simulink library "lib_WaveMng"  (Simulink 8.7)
settings: Solver=ode45  StartTime=0.0  StopTime=10.0  RelTol=1e-3
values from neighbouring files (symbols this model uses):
  Tstep = 0.0005    [TestOrthOscObjO_init.m]    (also in TestWaveMng_init.m = 5e-05)
undefined symbols (not defined in the file or in its folder): avgSteps, incrAvgSteps, P_WaveData_FB, P_WaveMng_FB, P_WaveMngIx_FB, stepA_WaveMngIx_FB, stepSimulink_AvgWave_FB, stepSimulink_WaveData_FB, stepSimulink_WaveMng_FB, u1, u2, void, work1, y1
libraries: lib_WaveMng x22, Lib_FunctionBlocks x6, lib_Conv x2

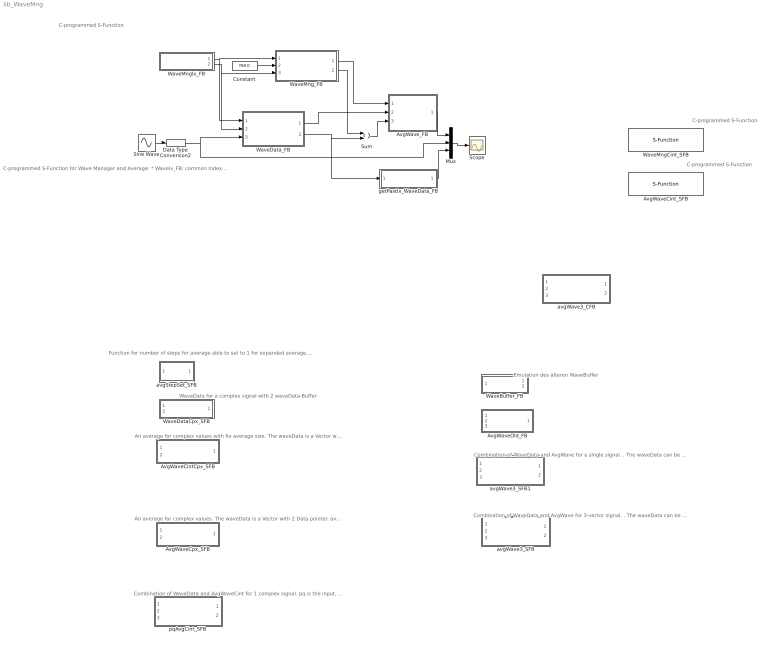
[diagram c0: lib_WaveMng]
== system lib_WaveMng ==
  note: Emulation des älteren WaveBuffer
  note: WaveData for a complex signal with 2 waveData-Buffer
  note: Function for number of steps for average able to set to 1 for expanded average. Parameter avgSteps
  note: C-programmed S-Function
  note: Combination of WaveData and AvgWaveCint for 1 complex signal. pq is the input, avg is the output. The waveData can be used for other accesses. It is a vector o2 2 pointer.
  note: An average for complex values. The waveData is a Vector with 2 Data pointer. avg is a complex output.
  note: C-programmed S-Function
  note: C-programmed S-Function
  note: C-programmed S-Function for Wave Manager and Average: * WaveIx_FB: common Index for one Buffer size. * WaveMng_FB: common manager for one average period but maybe more as one signal for averaging. * WaveData_FB; Buffer for data, for one signal value, but maybe for more as one average * AvgWave_FB: average for one signal and period. The connections ..._FB are references (ObjectOriented). The connections step... are only used to determine the calculation order.
  note: An average for complex values with fix average size. The waveData is a Vector with 2 Data pointer. avg is a complex output.
  note: Combination of WaveData and AvgWave for 3-vector signal. . The waveData can be used for other accesses. It is a vector o2 3 pointer.
  note: Combination of WaveData and AvgWave for a single signal. . The waveData can be used for other accesses. It is a pointer.
  AvgWaveCintCpx_SFB : Subsystem
  AvgWaveCint_SFB : S-Function  LoadFcn=defWaveMngPtr  FunctionName=AvgWaveCint_SFB  SFunctionDeploymentMode=off  EnableBusSupport=off
  AvgWaveCpx_SFB : Subsystem
  AvgWaveOld_FB : Subsystem
  AvgWave_FB : Subsystem
  Constant : Constant  Value=768.0  OutDataTypeStr=single
  Data Type Conversion2 : DataTypeConversion  OutDataTypeStr=single
  Mux : Mux  Inputs=3
  Scope : Scope
  Sine Wave : Sin  Amplitude=4  Frequency=10.02*pi  SampleTime=Tstep
  Sum : Sum
  WaveBuffer_FB : Subsystem
  WaveDataCpx_SFB : Subsystem
  WaveData_FB : Subsystem
  WaveMngCint_SFB : S-Function  FunctionName=WaveMngCint_SFB  SFunctionDeploymentMode=off  EnableBusSupport=off
  WaveMngIx_FB : Subsystem
  WaveMng_FB : Subsystem
  avgStepSet_SFB : Subsystem
  avgWave3_CFB : Subsystem
  avgWave3_SFB : Subsystem
  avgWave3_SFB1 : Subsystem
  getPastIx_WaveData_FB : Subsystem
  pqAvgCint_SFB : Subsystem
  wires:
  WaveMng_FB/1(Out1) -> AvgWave_FB/1(In2)
  Constant/1 -> WaveMng_FB/2(In3)
  Mux/1 -> Scope/1
  AvgWave_FB/1(Out2) -> Mux/1
  Sine Wave/1 -> Data Type Conversion2/1
  WaveMngIx_FB/1(Out1) -> WaveMng_FB/1(In2), WaveData_FB/1(In2)
  Data Type Conversion2/1 -> WaveData_FB/3(In3), Mux/2
  getPastIx_WaveData_FB/1(Out2) -> Mux/3
  WaveData_FB/1(Out1) -> AvgWave_FB/2(In4)
  WaveMngIx_FB/2(Out2) -> WaveData_FB/2(In1), WaveMng_FB/3(In1)
  WaveMng_FB/2(Out2) -> Sum/1
  WaveData_FB/2(Out2) -> getPastIx_WaveData_FB/1(In2), Sum/2
  Sum/1 -> AvgWave_FB/3(In1)

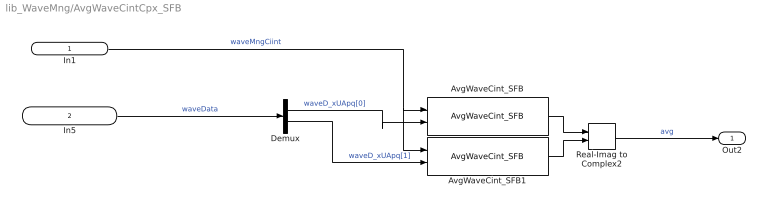
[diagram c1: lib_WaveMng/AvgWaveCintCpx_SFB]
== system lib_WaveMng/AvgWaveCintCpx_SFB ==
  In1 : Inport
  In5 : Inport  Port=2  OutDataTypeStr=P_WaveData_FB  PortDimensions=2
  AvgWaveCint_SFB : lib_WaveMng/AvgWaveCint_SFB  SFunctionSpec=stepSimulink_AvgWave_FB(void* work1, P_WaveMng_FB u1, P_WaveData_FB u2, single y1[1])  ShowSpec=off
  AvgWaveCint_SFB1 : lib_WaveMng/AvgWaveCint_SFB  SFunctionSpec=stepSimulink_AvgWave_FB(void* work1, P_WaveMng_FB u1, P_WaveData_FB u2, single y1[1])  ShowSpec=off
  Demux : Demux  Outputs=2
  Real-Imag to Complex2 : RealImagToComplex
  Out2 : Outport
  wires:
  In1/1 -> AvgWaveCint_SFB1/1, AvgWaveCint_SFB/1  "waveMngCiint"
  AvgWaveCint_SFB1/1 -> Real-Imag to Complex2/2
  Demux/1 -> AvgWaveCint_SFB/2  "waveD_xUApq[0]"
  AvgWaveCint_SFB/1 -> Real-Imag to Complex2/1
  In5/1 -> Demux/1  "waveData"
  Real-Imag to Complex2/1 -> Out2/1  "avg"
  Demux/2 -> AvgWaveCint_SFB1/2  "waveD_xUApq[1]"

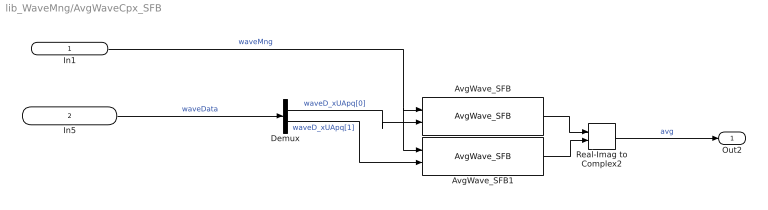
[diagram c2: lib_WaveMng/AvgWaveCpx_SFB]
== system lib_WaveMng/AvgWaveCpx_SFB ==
  In1 : Inport
  In5 : Inport  Port=2  OutDataTypeStr=P_WaveData_FB  PortDimensions=2
  AvgWave_SFB : Lib_FunctionBlocks/AvgWave_SFB  SFunctionSpec=stepSimulink_AvgWave_FB(void* work1, P_WaveMng_FB u1, P_WaveData_FB u2, single y1[1])  ShowSpec=off
  AvgWave_SFB1 : Lib_FunctionBlocks/AvgWave_SFB  SFunctionSpec=stepSimulink_AvgWave_FB(void* work1, P_WaveMng_FB u1, P_WaveData_FB u2, single y1[1])  ShowSpec=off
  Demux : Demux  Outputs=2
  Real-Imag to Complex2 : RealImagToComplex
  Out2 : Outport
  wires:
  In1/1 -> AvgWave_SFB1/1, AvgWave_SFB/1  "waveMng"
  AvgWave_SFB1/1 -> Real-Imag to Complex2/2
  Demux/1 -> AvgWave_SFB/2  "waveD_xUApq[0]"
  AvgWave_SFB/1 -> Real-Imag to Complex2/1
  In5/1 -> Demux/1  "waveData"
  Real-Imag to Complex2/1 -> Out2/1  "avg"
  Demux/2 -> AvgWave_SFB1/2  "waveD_xUApq[1]"

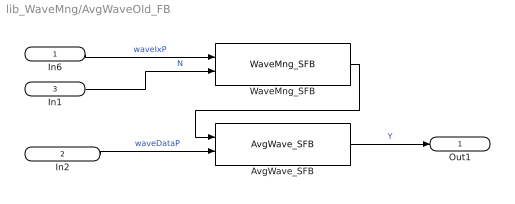
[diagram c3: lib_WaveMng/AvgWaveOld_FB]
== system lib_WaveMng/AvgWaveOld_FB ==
  In6 : Inport  OutDataTypeStr=P_WaveMngIx_FB
  In2 : Inport  Port=2  OutDataTypeStr=P_WaveData_FB
  In1 : Inport  Port=3  OutDataTypeStr=P_WaveMngIx_FB  PortDimensions=1
  AvgWave_SFB : lib_WaveMng/AvgWave_SFB  SFunctionSpec=stepSimulink_AvgWave_FB(void* work1, P_WaveMng_FB u1, P_WaveData_FB u2, single y1[1])  ShowSpec=off
  WaveMng_SFB : lib_WaveMng/WaveMng_SFB  SFunctionSpec=stepSimulink_WaveMng_FB(void* work1, P_WaveMngIx_FB u1, single u2, P_WaveMng_FB y1[1])  ShowSpec=off
  Out1 : Outport  OutDataTypeStr=single
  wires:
  WaveMng_SFB/1 -> AvgWave_SFB/1
  In6/1 -> WaveMng_SFB/1  "waveIxP"
  In1/1 -> WaveMng_SFB/2  "N"
  In2/1 -> AvgWave_SFB/2  "waveDataP"
  AvgWave_SFB/1 -> Out1/1  "Y"

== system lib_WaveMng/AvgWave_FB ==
  In2 : Inport  OutDataTypeStr=uint32
  In4 : Inport  Port=2  OutDataTypeStr=uint32
  In1 : Inport  Port=3  OutDataTypeStr=uint32
  AvgWave_SFB : S-Function  LoadFcn=defWaveMngPtr  FunctionName=step_AvgWave_FB_SfH  Parameters=123  SFunctionDeploymentMode=off  EnableBusSupport=off
  Out2 : Outport  OutDataTypeStr=single
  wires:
  In4/1 -> AvgWave_SFB/2  "WaveData"
  In2/1 -> AvgWave_SFB/1  "WaveMng_FB"
  AvgWave_SFB/2 -> Out2/1  "avg"
  In1/1 -> AvgWave_SFB/3  "step"

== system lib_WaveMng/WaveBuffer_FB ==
  In9 : Inport  OutDataTypeStr=single  PortDimensions=1
  WaveData_SFB : lib_WaveMng/WaveData_SFB  SFunctionSpec=stepSimulink_WaveData_FB(void* work1, P_WaveMngIx_FB u1, single u2, P_WaveData_FB y1[1])  ShowSpec=off
  WaveMngIx_SFB : lib_WaveMng/WaveMngIx_SFB  SFunctionSpec=stepA_WaveMngIx_FB(void* work1, P_WaveMngIx_FB y1[1])  SParameter1=1024  ShowSpec=off
  Out3 : Outport  OutDataTypeStr=P_WaveData_FB  PortDimensions=1
  Out1 : Outport  Port=2  OutDataTypeStr=P_WaveMngIx_FB  PortDimensions=1
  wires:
  WaveMngIx_SFB/1 -> Out1/1, WaveData_SFB/1  "waveIxP"
  In9/1 -> WaveData_SFB/2  "X"
  WaveData_SFB/1 -> Out3/1  "WaveData"

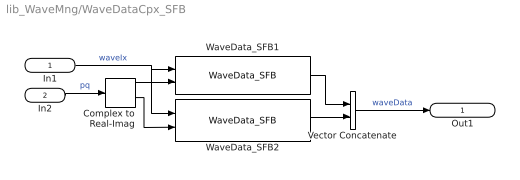
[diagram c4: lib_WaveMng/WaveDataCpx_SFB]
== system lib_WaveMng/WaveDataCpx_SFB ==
  In1 : Inport
  In2 : Inport  Port=2
  Complex to Real-Imag : ComplexToRealImag
  Vector Concatenate : Concatenate
  WaveData_SFB1 : lib_WaveMng/WaveData_SFB  SFunctionSpec=stepSimulink_WaveData_FB(void* work1, P_WaveMngIx_FB u1, single u2, P_WaveData_FB y1[1])  ShowSpec=off
  WaveData_SFB2 : lib_WaveMng/WaveData_SFB  SFunctionSpec=stepSimulink_WaveData_FB(void* work1, P_WaveMngIx_FB u1, single u2, P_WaveData_FB y1[1])  ShowSpec=off
  Out1 : Outport
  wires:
  Complex to Real-Imag/2 -> WaveData_SFB2/2
  In1/1 -> WaveData_SFB2/1, WaveData_SFB1/1  "waveIx"
  Complex to Real-Imag/1 -> WaveData_SFB1/2
  In2/1 -> Complex to Real-Imag/1  "pq"
  Vector Concatenate/1 -> Out1/1  "waveData"
  WaveData_SFB2/1 -> Vector Concatenate/2
  WaveData_SFB1/1 -> Vector Concatenate/1

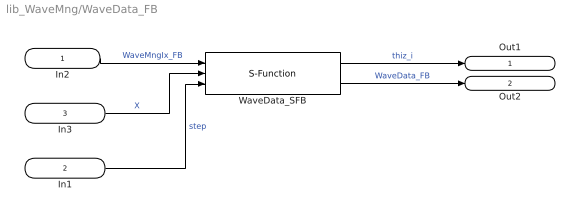
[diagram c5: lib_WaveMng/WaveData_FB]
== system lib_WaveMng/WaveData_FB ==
  In2 : Inport  OutDataTypeStr=uint32
  In1 : Inport  Port=2  OutDataTypeStr=uint32
  In3 : Inport  Port=3  OutDataTypeStr=single
  WaveData_SFB : S-Function  FunctionName=step_WaveData_FB_SfH  Parameters=123 1024  SFunctionDeploymentMode=off  EnableBusSupport=off
  Out1 : Outport  OutDataTypeStr=uint32
  Out2 : Outport  Port=2  OutDataTypeStr=uint32
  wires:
  In3/1 -> WaveData_SFB/2  "X"
  In2/1 -> WaveData_SFB/1  "WaveMngIx_FB"
  WaveData_SFB/1 -> Out1/1  "thiz_i"
  WaveData_SFB/2 -> Out2/1  "WaveData_FB"
  In1/1 -> WaveData_SFB/3  "step"

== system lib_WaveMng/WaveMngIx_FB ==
  WaveMngIx_FB : S-Function  FunctionName=step_WaveMngIx_FB_SfH  Parameters=identObj size Tstep  SFunctionDeploymentMode=off  EnableBusSupport=off
  Out1 : Outport  OutDataTypeStr=uint32
  Out2 : Outport  Port=2  OutDataTypeStr=uint32
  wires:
  WaveMngIx_FB/1 -> Out1/1  "WaveMngIx_FB"
  WaveMngIx_FB/2 -> Out2/1  "step"

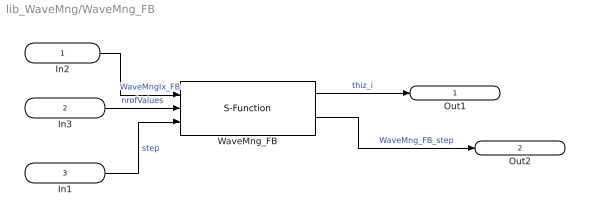
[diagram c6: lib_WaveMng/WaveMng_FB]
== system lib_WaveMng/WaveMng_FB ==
  In2 : Inport  OutDataTypeStr=uint32
  In3 : Inport  Port=2  OutDataTypeStr=single
  In1 : Inport  Port=3  OutDataTypeStr=uint32
  WaveMng_FB : S-Function  FunctionName=step_WaveMng_FB_SfH  Parameters=identObj  SFunctionDeploymentMode=off  EnableBusSupport=off
  Out1 : Outport  OutDataTypeStr=uint32
  Out2 : Outport  Port=2  OutDataTypeStr=uint32
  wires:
  WaveMng_FB/1 -> Out1/1  "thiz_i"
  In2/1 -> WaveMng_FB/1  "WaveMngIx_FB"
  In3/1 -> WaveMng_FB/2  "nrofValues"
  In1/1 -> WaveMng_FB/3  "step"
  WaveMng_FB/2 -> Out2/1  "WaveMng_FB_step"

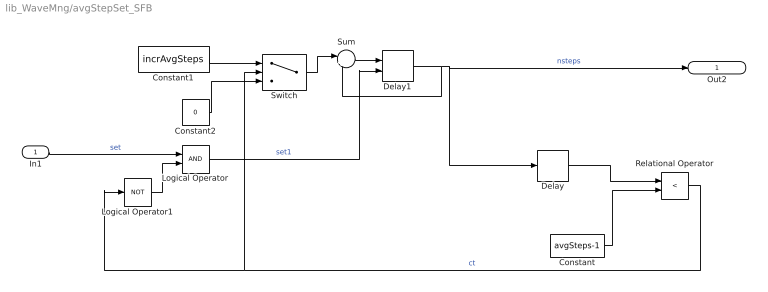
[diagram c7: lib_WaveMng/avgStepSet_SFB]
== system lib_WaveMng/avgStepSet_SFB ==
  In1 : Inport
  Constant : Constant  Value=avgSteps-1  OutDataTypeStr=single
  Constant1 : Constant  Value=incrAvgSteps  OutDataTypeStr=single
  Constant2 : Constant  Value=0  OutDataTypeStr=single
  Delay : Delay  DelayLength=1
  Delay1 : Delay  DelayLength=1  InitialCondition=1.0  ExternalReset=Level
  Logical Operator : Logic  AllPortsSameDT=off  OutDataTypeStr=boolean
  Logical Operator1 : Logic  Operator=NOT  AllPortsSameDT=off  OutDataTypeStr=boolean
  Relational Operator : RelationalOperator  Operator=<  OutDataTypeStr=boolean
  Sum : Sum  Inputs=|++
  Switch : Switch  Criteria=u2 ~= 0
  Out2 : Outport  OutDataTypeStr=single
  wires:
  Delay1/1 -> Delay/1, Out2/1, Sum/2  "nsteps"
  Constant/1 -> Relational Operator/2
  Delay/1 -> Relational Operator/1
  Sum/1 -> Delay1/1
  Constant1/1 -> Switch/1
  Logical Operator/1 -> Delay1/2  "set1"
  Switch/1 -> Sum/1
  Constant2/1 -> Switch/3
  Relational Operator/1 -> Logical Operator1/1, Switch/2  "ct"
  In1/1 -> Logical Operator/1  "set"
  Logical Operator1/1 -> Logical Operator/2

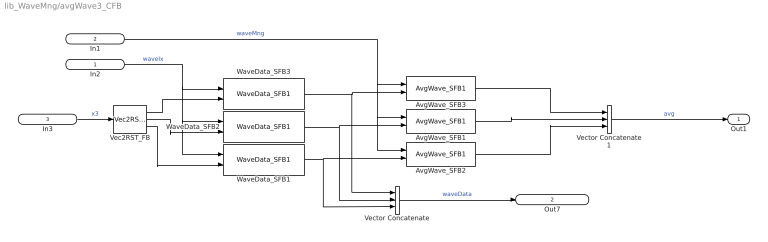
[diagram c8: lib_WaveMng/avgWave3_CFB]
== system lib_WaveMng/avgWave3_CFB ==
  In2 : Inport  OutDataTypeStr=Bus: WaveMngIx_FB
  In1 : Inport  Port=2  OutDataTypeStr=Bus: WaveMng_FB
  In3 : Inport  Port=3  OutDataTypeStr=single  PortDimensions=3
  AvgWave_SFB1 : lib_WaveMng/AvgWave_SFB1  SFunctionSpec=stepSimulink_AvgWave_FB(void* work1, P_WaveMng_FB u1, P_WaveData_FB u2, single y1[1])  ShowSpec=off
  AvgWave_SFB2 : lib_WaveMng/AvgWave_SFB1  SFunctionSpec=stepSimulink_AvgWave_FB(void* work1, P_WaveMng_FB u1, P_WaveData_FB u2, single y1[1])  ShowSpec=off
  AvgWave_SFB3 : lib_WaveMng/AvgWave_SFB1  SFunctionSpec=stepSimulink_AvgWave_FB(void* work1, P_WaveMng_FB u1, P_WaveData_FB u2, single y1[1])  ShowSpec=off
  Vec2RST_FB : lib_Conv/Vec2RST_FB
  Vector Concatenate : Concatenate  NumInputs=3
  Vector Concatenate1 : Concatenate  NumInputs=3
  WaveData_SFB1 : lib_WaveMng/WaveData_SFB1  SFunctionSpec=stepSimulink_WaveData_FB(void* work1, P_WaveMngIx_FB u1, single u2, P_WaveData_FB y1[1])  ShowSpec=off
  WaveData_SFB2 : lib_WaveMng/WaveData_SFB1  SFunctionSpec=stepSimulink_WaveData_FB(void* work1, P_WaveMngIx_FB u1, single u2, P_WaveData_FB y1[1])  ShowSpec=off
  WaveData_SFB3 : lib_WaveMng/WaveData_SFB1  SFunctionSpec=stepSimulink_WaveData_FB(void* work1, P_WaveMngIx_FB u1, single u2, P_WaveData_FB y1[1])  ShowSpec=off
  Out1 : Outport  OutDataTypeStr=single  PortDimensions=3
  Out7 : Outport  Port=2  OutDataTypeStr=Bus: WaveData_FB  PortDimensions=3
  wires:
  AvgWave_SFB2/1 -> Vector Concatenate1/3
  WaveData_SFB1/1 -> AvgWave_SFB2/2, Vector Concatenate/3
  Vec2RST_FB/3 -> WaveData_SFB1/2
  AvgWave_SFB1/1 -> Vector Concatenate1/2
  AvgWave_SFB3/1 -> Vector Concatenate1/1
  Vec2RST_FB/2 -> WaveData_SFB2/2
  WaveData_SFB2/1 -> AvgWave_SFB1/2, Vector Concatenate/2
  In2/1 -> WaveData_SFB3/1, WaveData_SFB1/1, WaveData_SFB2/1  "waveIx"
  WaveData_SFB3/1 -> AvgWave_SFB3/2, Vector Concatenate/1
  In1/1 -> AvgWave_SFB2/1, AvgWave_SFB1/1, AvgWave_SFB3/1  "waveMng"
  Vec2RST_FB/1 -> WaveData_SFB3/2
  Vector Concatenate1/1 -> Out1/1  "avg"
  In3/1 -> Vec2RST_FB/1  "x3"
  Vector Concatenate/1 -> Out7/1  "waveData"

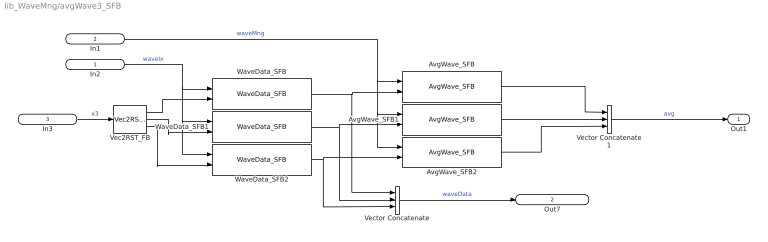
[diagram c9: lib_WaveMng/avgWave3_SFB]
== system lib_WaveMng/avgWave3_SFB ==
  In2 : Inport  OutDataTypeStr=P_WaveMngIx_FB
  In1 : Inport  Port=2  OutDataTypeStr=P_WaveMngCint_FB
  In3 : Inport  Port=3  OutDataTypeStr=single  PortDimensions=3
  AvgWave_SFB : lib_WaveMng/AvgWave_SFB  SFunctionSpec=stepSimulink_AvgWave_FB(void* work1, P_WaveMng_FB u1, P_WaveData_FB u2, single y1[1])  ShowSpec=off
  AvgWave_SFB1 : lib_WaveMng/AvgWave_SFB  SFunctionSpec=stepSimulink_AvgWave_FB(void* work1, P_WaveMng_FB u1, P_WaveData_FB u2, single y1[1])  ShowSpec=off
  AvgWave_SFB2 : lib_WaveMng/AvgWave_SFB  SFunctionSpec=stepSimulink_AvgWave_FB(void* work1, P_WaveMng_FB u1, P_WaveData_FB u2, single y1[1])  ShowSpec=off
  Vec2RST_FB : lib_Conv/Vec2RST_FB
  Vector Concatenate : Concatenate  NumInputs=3
  Vector Concatenate1 : Concatenate  NumInputs=3
  WaveData_SFB : lib_WaveMng/WaveData_SFB  SFunctionSpec=stepSimulink_WaveData_FB(void* work1, P_WaveMngIx_FB u1, single u2, P_WaveData_FB y1[1])  ShowSpec=off
  WaveData_SFB1 : lib_WaveMng/WaveData_SFB  SFunctionSpec=stepSimulink_WaveData_FB(void* work1, P_WaveMngIx_FB u1, single u2, P_WaveData_FB y1[1])  ShowSpec=off
  WaveData_SFB2 : lib_WaveMng/WaveData_SFB  SFunctionSpec=stepSimulink_WaveData_FB(void* work1, P_WaveMngIx_FB u1, single u2, P_WaveData_FB y1[1])  ShowSpec=off
  Out1 : Outport  OutDataTypeStr=single  PortDimensions=3
  Out7 : Outport  Port=2  OutDataTypeStr=P_WaveData_FB  PortDimensions=3
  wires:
  Vector Concatenate/1 -> Out7/1  "waveData"
  In3/1 -> Vec2RST_FB/1  "x3"
  Vector Concatenate1/1 -> Out1/1  "avg"
  Vec2RST_FB/1 -> WaveData_SFB/2
  In1/1 -> AvgWave_SFB/1, AvgWave_SFB2/1, AvgWave_SFB1/1  "waveMng"
  WaveData_SFB/1 -> Vector Concatenate/1, AvgWave_SFB/2
  In2/1 -> WaveData_SFB/1, WaveData_SFB2/1, WaveData_SFB1/1  "waveIx"
  WaveData_SFB1/1 -> Vector Concatenate/2, AvgWave_SFB1/2
  Vec2RST_FB/2 -> WaveData_SFB1/2
  AvgWave_SFB/1 -> Vector Concatenate1/1
  AvgWave_SFB1/1 -> Vector Concatenate1/2
  Vec2RST_FB/3 -> WaveData_SFB2/2
  WaveData_SFB2/1 -> Vector Concatenate/3, AvgWave_SFB2/2
  AvgWave_SFB2/1 -> Vector Concatenate1/3

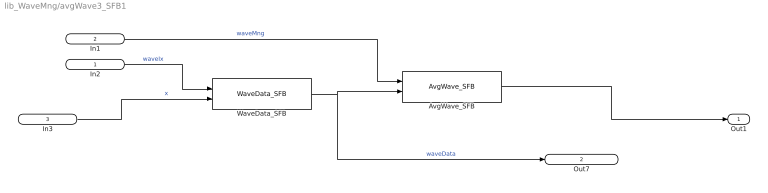
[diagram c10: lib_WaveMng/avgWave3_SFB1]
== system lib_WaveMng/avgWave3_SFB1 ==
  In2 : Inport  OutDataTypeStr=P_WaveMngIx_FB
  In1 : Inport  Port=2  OutDataTypeStr=P_WaveMngCint_FB
  In3 : Inport  Port=3  OutDataTypeStr=single  PortDimensions=1
  AvgWave_SFB : lib_WaveMng/AvgWave_SFB  SFunctionSpec=stepSimulink_AvgWave_FB(void* work1, P_WaveMng_FB u1, P_WaveData_FB u2, single y1[1])  ShowSpec=off
  WaveData_SFB : lib_WaveMng/WaveData_SFB  SFunctionSpec=stepSimulink_WaveData_FB(void* work1, P_WaveMngIx_FB u1, single u2, P_WaveData_FB y1[1])  ShowSpec=off
  Out1 : Outport  OutDataTypeStr=single  PortDimensions=1
  Out7 : Outport  Port=2  OutDataTypeStr=P_WaveData_FB  PortDimensions=1
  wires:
  AvgWave_SFB/1 -> Out1/1
  In2/1 -> WaveData_SFB/1  "waveIx"
  In1/1 -> AvgWave_SFB/1  "waveMng"
  In3/1 -> WaveData_SFB/2  "x"
  WaveData_SFB/1 -> Out7/1, AvgWave_SFB/2  "waveData"

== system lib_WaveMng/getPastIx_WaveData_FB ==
  In2 : Inport  OutDataTypeStr=uint32
  getPastIx_WaveData_SFB : S-Function  FunctionName=getPastIx_WaveData_FB_SfH  Parameters=ixPast  SFunctionDeploymentMode=off  EnableBusSupport=off
  Out2 : Outport  OutDataTypeStr=single
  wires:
  In2/1 -> getPastIx_WaveData_SFB/1  "WaveData_FB"
  getPastIx_WaveData_SFB/1 -> Out2/1  "past"

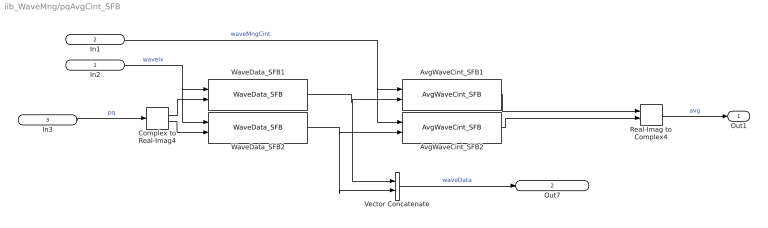
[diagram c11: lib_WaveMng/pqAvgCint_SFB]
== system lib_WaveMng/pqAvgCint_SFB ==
  In2 : Inport  OutDataTypeStr=P_WaveMngIx_FB
  In1 : Inport  Port=2  OutDataTypeStr=P_WaveMngCint_FB
  In3 : Inport  Port=3  OutDataTypeStr=single
  AvgWaveCint_SFB1 : Lib_FunctionBlocks/AvgWaveCint_SFB  SFunctionSpec=stepSimulink_AvgWave_FB(void* work1, P_WaveMng_FB u1, P_WaveData_FB u2, single y1[1])  ShowSpec=off
  AvgWaveCint_SFB2 : Lib_FunctionBlocks/AvgWaveCint_SFB  SFunctionSpec=stepSimulink_AvgWave_FB(void* work1, P_WaveMng_FB u1, P_WaveData_FB u2, single y1[1])  ShowSpec=off
  Complex to Real-Imag4 : ComplexToRealImag
  Real-Imag to Complex4 : RealImagToComplex
  Vector Concatenate : Concatenate
  WaveData_SFB1 : Lib_FunctionBlocks/WaveData_SFB  SFunctionSpec=stepSimulink_WaveData_FB(void* work1, P_WaveMngIx_FB u1, single u2, P_WaveData_FB y1[1])  ShowSpec=off
  WaveData_SFB2 : Lib_FunctionBlocks/WaveData_SFB  SFunctionSpec=stepSimulink_WaveData_FB(void* work1, P_WaveMngIx_FB u1, single u2, P_WaveData_FB y1[1])  ShowSpec=off
  Out1 : Outport  OutDataTypeStr=single
  Out7 : Outport  Port=2  OutDataTypeStr=P_WaveData_FB  PortDimensions=2
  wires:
  AvgWaveCint_SFB2/1 -> Real-Imag to Complex4/2
  AvgWaveCint_SFB1/1 -> Real-Imag to Complex4/1
  Complex to Real-Imag4/2 -> WaveData_SFB2/2
  WaveData_SFB2/1 -> Vector Concatenate/2, AvgWaveCint_SFB2/2
  In2/1 -> WaveData_SFB2/1, WaveData_SFB1/1  "waveIx"
  WaveData_SFB1/1 -> Vector Concatenate/1, AvgWaveCint_SFB1/2
  In1/1 -> AvgWaveCint_SFB2/1, AvgWaveCint_SFB1/1  "waveMngCint"
  Complex to Real-Imag4/1 -> WaveData_SFB1/2
  Real-Imag to Complex4/1 -> Out1/1  "avg"
  In3/1 -> Complex to Real-Imag4/1  "pq"
  Vector Concatenate/1 -> Out7/1  "waveData"
